(* Logix 5000 AddOnInstructionDefinition export SPEL_Above; software revision 30.01; part 6 of 9 *)

ADD_ON_INSTRUCTION SPEL_MotorGet   (* revision 1.2, vendor SEIKO EPSON CORP. *)
// Gets the state of the motor.
VAR_INPUT
   Start : BOOL; {required}
END_VAR
VAR_OUTPUT
   InCycle : BOOL; {access None, visible}
END_VAR
VAR_IN_OUT
   ExtInputs : AB:ETHERNET_MODULE_INT_128Bytes:I:0; {required}
   ExtOutputs : AB:ETHERNET_MODULE_INT_128Bytes:O:0; {required}
END_VAR
VAR_OUTPUT
   ErrCode1 : INT; {access None, visible}
   ErrCode2 : INT; {access None, visible}
   Status : INT; {visible}
   Done : BOOL; {access Read Only, visible}
   Error : BOOL; {visible}
END_VAR
VAR
   ExecMotor : SPEL_ExecCmd := (MaxTime := 3000); {access None}
   ExecTimeout : DINT; {access None}
END_VAR

ROUTINE Logic   (* ladder *)
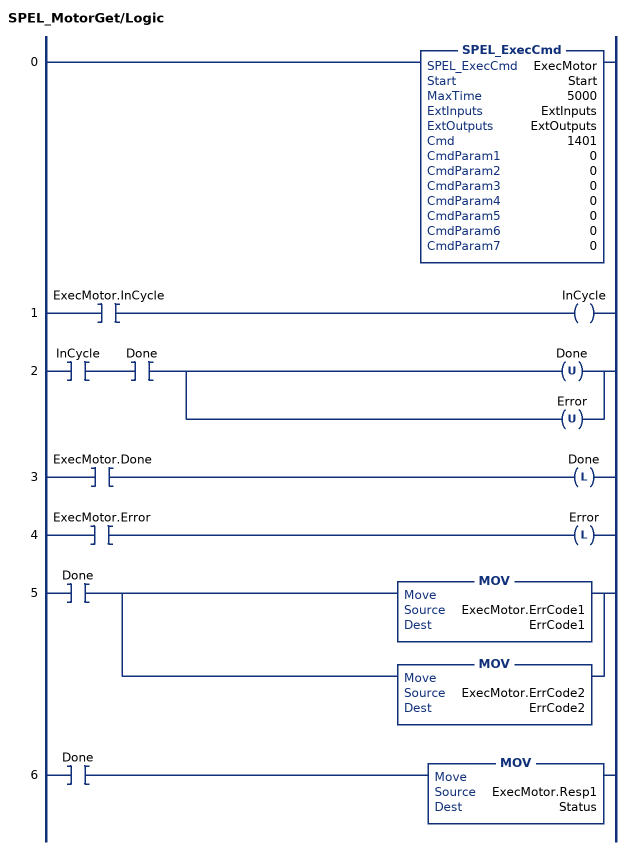
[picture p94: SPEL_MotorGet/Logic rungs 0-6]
   0: SPEL_ExecCmd(ExecMotor,Start,5000,ExtInputs,ExtOutputs,1401,0,0,0,0,0,0,0);
   1: XIC(ExecMotor.InCycle)OTE(InCycle);
   2: XIC(InCycle)XIC(Done)[OTU(Done) ,OTU(Error) ];
   3: XIC(ExecMotor.Done)OTL(Done);
   4: XIC(ExecMotor.Error)OTL(Error);
   5: XIC(Done)[MOV(ExecMotor.ErrCode1,ErrCode1) ,MOV(ExecMotor.ErrCode2,ErrCode2) ];
   6: XIC(Done)MOV(ExecMotor.Resp1,Status);
END_ROUTINE
END_ADD_ON_INSTRUCTION

ADD_ON_INSTRUCTION SPEL_MotorOff   (* revision 1.0, vendor SEIKO EPSON CORP. *)
// Turns robot motors off.
VAR_INPUT
   Start : BOOL; {access Read Only, required}
END_VAR
VAR_OUTPUT
   InCycle : BOOL; {access Read Only, visible}
   Done : BOOL; {access Read Only, visible}
   Error : BOOL; {access Read Only, visible}
END_VAR
VAR_IN_OUT
   ExtInputs : AB:ETHERNET_MODULE_INT_128Bytes:I:0; {required}
   ExtOutputs : AB:ETHERNET_MODULE_INT_128Bytes:O:0; {required}
END_VAR
VAR_OUTPUT
   ErrCode1 : INT; {access Read Only, visible}
   ErrCode2 : INT; {access Read Only, visible}
END_VAR
VAR
   ExecMotorOff : SPEL_ExecCmd := (MaxTime := 3000); {access None}
        .INCYCLE   // ExecInCycle
        .DONE   // ExecDone
        .ERROR   // ExecError
   OneShotStart : BOOL; {access None}
   StartCoil : BOOL; {access None}
   ExecTimeout : DINT; {access None}
END_VAR

ROUTINE Logic   (* ladder *)
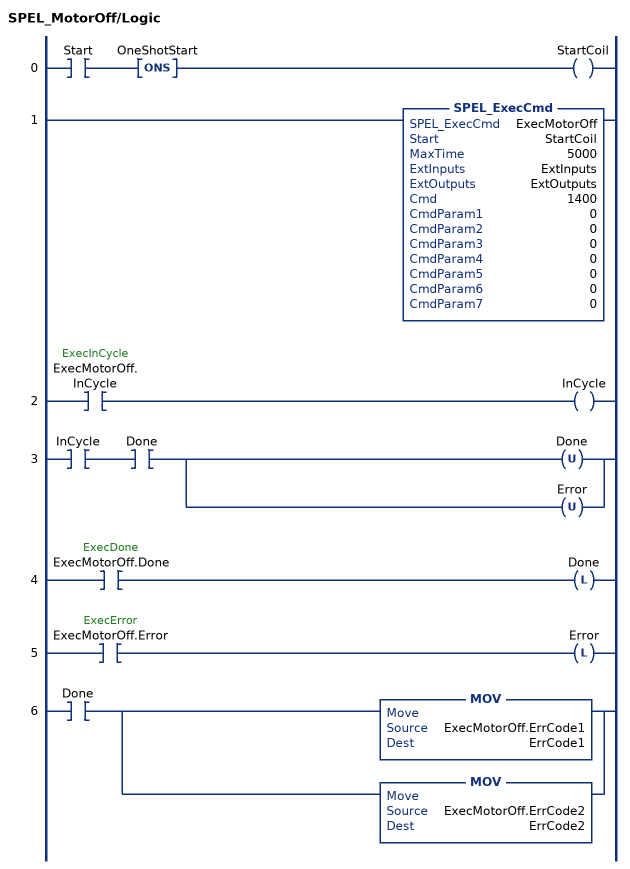
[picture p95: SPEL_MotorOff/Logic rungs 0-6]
   0: XIC(Start)ONS(OneShotStart)OTE(StartCoil);
   1: SPEL_ExecCmd(ExecMotorOff,StartCoil,5000,ExtInputs,ExtOutputs,1400,0,0,0,0,0,0,0);
   2: XIC(ExecMotorOff.InCycle)OTE(InCycle);
   3: XIC(InCycle)XIC(Done)[OTU(Done) ,OTU(Error) ];
   4: XIC(ExecMotorOff.Done)OTL(Done);
   5: XIC(ExecMotorOff.Error)OTL(Error);
   6: XIC(Done)[MOV(ExecMotorOff.ErrCode1,ErrCode1) ,MOV(ExecMotorOff.ErrCode2,ErrCode2) ];
END_ROUTINE
END_ADD_ON_INSTRUCTION

ADD_ON_INSTRUCTION SPEL_MotorOn   (* revision 1.0, vendor SEIKO EPSON CORP. *)
// Turns robot motors on.
VAR_INPUT
   Start : BOOL; {access Read Only, required}
END_VAR
VAR_OUTPUT
   InCycle : BOOL; {access Read Only, visible}
   Done : BOOL; {access Read Only, visible}
   Error : BOOL; {access Read Only, visible}
END_VAR
VAR_IN_OUT
   ExtInputs : AB:ETHERNET_MODULE_INT_128Bytes:I:0; {required}
   ExtOutputs : AB:ETHERNET_MODULE_INT_128Bytes:O:0; {required}
END_VAR
VAR_OUTPUT
   ErrCode1 : INT; {access Read Only, visible}
   ErrCode2 : INT; {access Read Only, visible}
END_VAR
VAR
   ExecMotorOn : SPEL_ExecCmd := (MaxTime := 3000); {access None}
        .INCYCLE   // ExecInCycle
        .DONE   // ExecDone
        .ERROR   // ExecError
   OneShotStart : BOOL; {access None}
   StartCoil : BOOL; {access None}
   ExecTimeout : DINT; {access None}
END_VAR

ROUTINE Logic   (* ladder *)
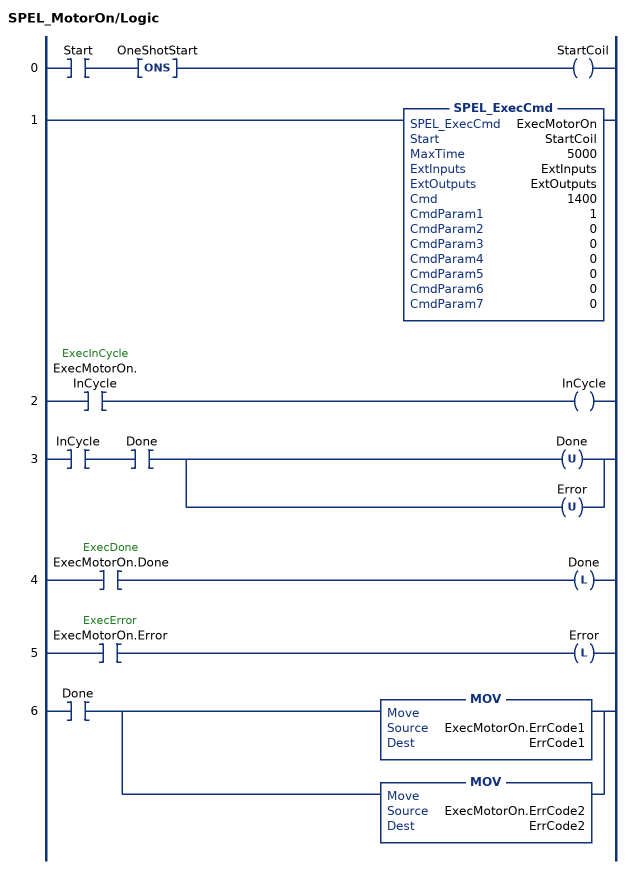
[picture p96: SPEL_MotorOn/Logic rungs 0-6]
   0: XIC(Start)ONS(OneShotStart)OTE(StartCoil);
   1: SPEL_ExecCmd(ExecMotorOn,StartCoil,5000,ExtInputs,ExtOutputs,1400,1,0,0,0,0,0,0);
   2: XIC(ExecMotorOn.InCycle)OTE(InCycle);
   3: XIC(InCycle)XIC(Done)[OTU(Done) ,OTU(Error) ];
   4: XIC(ExecMotorOn.Done)OTL(Done);
   5: XIC(ExecMotorOn.Error)OTL(Error);
   6: XIC(Done)[MOV(ExecMotorOn.ErrCode1,ErrCode1) ,MOV(ExecMotorOn.ErrCode2,ErrCode2) ];
END_ROUTINE
END_ADD_ON_INSTRUCTION

ADD_ON_INSTRUCTION SPEL_Move   (* revision 1.0, vendor SEIKO EPSON CORP. *)
// Moves the arm from the current position to the specified position in a linear interpolation motion.
VAR_OUTPUT
   InCycle : BOOL; {access Read Only, visible}
   Done : BOOL; {access Read Only, visible}
   Error : BOOL; {access Read Only, visible}
END_VAR
VAR_INPUT
   Start : BOOL; {required}
   MaxTime : DINT := 30000; {access None, visible}
   TargetType : INT; {access None, visible}
   Point : INT; {required}
   PalletNum : INT; {access None, visible}
   PalletPosOrCol : INT; {access None, visible}
   PalletRow : INT; {access None, visible}
END_VAR
VAR_IN_OUT
   ExtInputs : AB:ETHERNET_MODULE_INT_128Bytes:I:0; {required}
   ExtOutputs : AB:ETHERNET_MODULE_INT_128Bytes:O:0; {required}
END_VAR
VAR_OUTPUT
   ErrCode1 : INT; {access Read Only, visible}
   ErrCode2 : INT; {access Read Only, visible}
END_VAR
VAR
   ExecMove : SPEL_ExecCmd := (MaxTime := 3000); {access None}
   StartInit : BOOL; {access None}
   PointOrPalletNum : INT; {access None}
   MoveTargetType : DINT; {access None}
   OneShotStart : BOOL; {access None}
   ExecTimeout : DINT; {access None}
   OneShotCP : BOOL; {access None}
   LocalCP : DINT; {access None}
   CmdParam1 : DINT; {access None}
   TargetTypeError : BOOL; {access None}
   StartExec : BOOL; {access None}
   ExecuteCmd : BOOL; {access None}
   OneShotTargetType : BOOL; {access None}
END_VAR

ROUTINE Logic   (* ladder *)
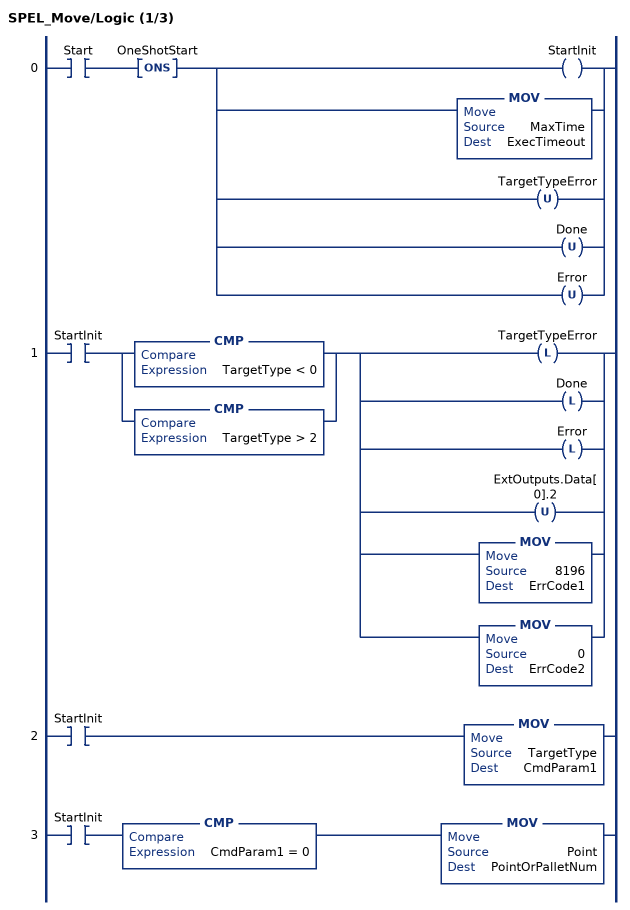
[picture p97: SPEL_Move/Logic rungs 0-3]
   0: XIC(Start)ONS(OneShotStart)[OTE(StartInit) ,MOV(MaxTime,ExecTimeout) ,OTU(TargetTypeError) ,OTU(Done) ,OTU(Error) ];
   1: XIC(StartInit)[CMP(TargetType < 0) ,CMP(TargetType > 2) ][OTL(TargetTypeError) ,OTL(Done) ,OTL(Error) ,OTU(ExtOutputs.Data[0].2) ,MOV(8196,ErrCode1) ,MOV(0,ErrCode2) ];
   2: XIC(StartInit)MOV(TargetType,CmdParam1);
   3: XIC(StartInit)CMP(CmdParam1 = 0)MOV(Point,PointOrPalletNum);
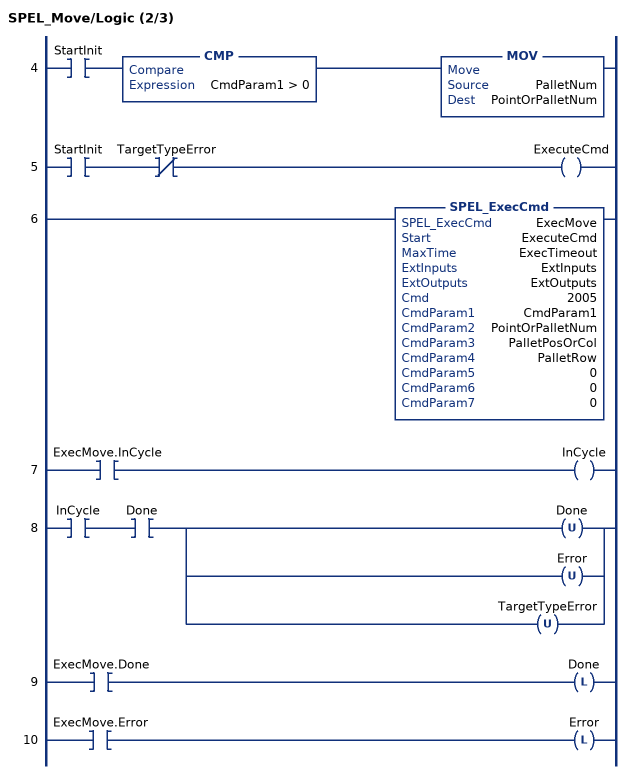
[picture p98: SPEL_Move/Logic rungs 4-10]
   4: XIC(StartInit)CMP(CmdParam1 > 0)MOV(PalletNum,PointOrPalletNum);
   5: XIC(StartInit)XIO(TargetTypeError)OTE(ExecuteCmd);
   6: SPEL_ExecCmd(ExecMove,ExecuteCmd,ExecTimeout,ExtInputs,ExtOutputs,2005,CmdParam1,PointOrPalletNum,PalletPosOrCol,PalletRow,0,0,0);
   7: XIC(ExecMove.InCycle)OTE(InCycle);
   8: XIC(InCycle)XIC(Done)[OTU(Done) ,OTU(Error) ,OTU(TargetTypeError) ];
   9: XIC(ExecMove.Done)OTL(Done);
   10: XIC(ExecMove.Error)OTL(Error);
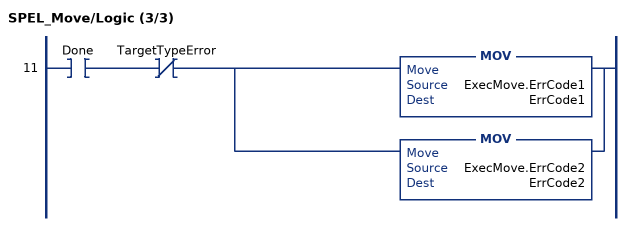
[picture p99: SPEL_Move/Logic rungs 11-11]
   11: XIC(Done)XIO(TargetTypeError)[MOV(ExecMove.ErrCode1,ErrCode1) ,MOV(ExecMove.ErrCode2,ErrCode2) ];
END_ROUTINE
END_ADD_ON_INSTRUCTION

ADD_ON_INSTRUCTION SPEL_NoFlip   (* revision 1.0, vendor SEIKO EPSON CORP. *)
// Sets the wrist orientation of the specified point to NOFLIP.
VAR_OUTPUT
   InCycle : BOOL; {access Read Only, visible}
   Done : BOOL; {access Read Only, visible}
   Error : BOOL; {access Read Only, visible}
END_VAR
VAR_INPUT
   Start : BOOL; {required}
   Point : INT; {required}
END_VAR
VAR_IN_OUT
   ExtInputs : AB:ETHERNET_MODULE_INT_128Bytes:I:0; {required}
   ExtOutputs : AB:ETHERNET_MODULE_INT_128Bytes:O:0; {required}
END_VAR
VAR_OUTPUT
   ErrCode1 : INT; {access Read Only, visible}
   ErrCode2 : INT; {access Read Only, visible}
END_VAR
VAR
   ExecNoFlip : SPEL_ExecCmd := (MaxTime := 3000); {access None}
   OneShotStart : BOOL; {access None}
   StartCoil : BOOL; {access None}
   ExecTimeout : DINT; {access None}
END_VAR

ROUTINE Logic   (* ladder *)
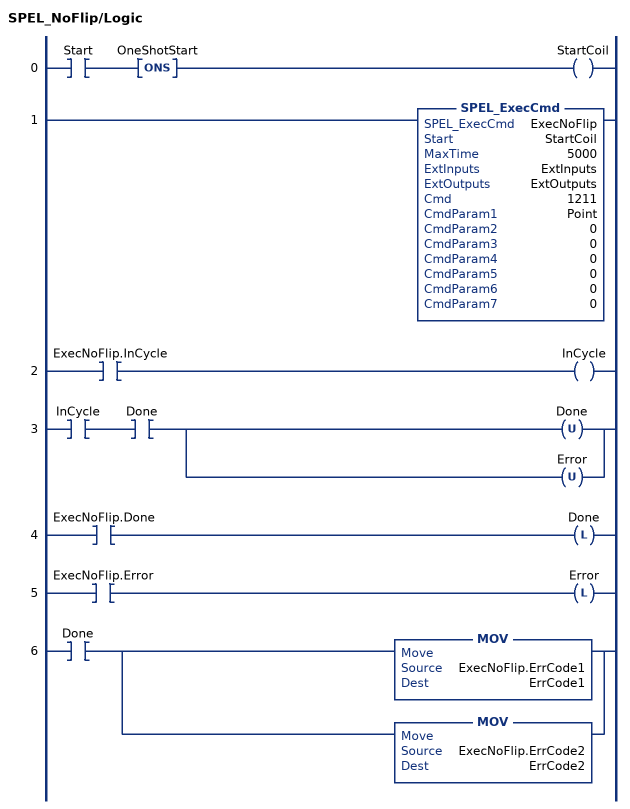
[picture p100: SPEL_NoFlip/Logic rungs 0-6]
   0: XIC(Start)ONS(OneShotStart)OTE(StartCoil);
   1: SPEL_ExecCmd(ExecNoFlip,StartCoil,5000,ExtInputs,ExtOutputs,1211,Point,0,0,0,0,0,0);
   2: XIC(ExecNoFlip.InCycle)OTE(InCycle);
   3: XIC(InCycle)XIC(Done)[OTU(Done) ,OTU(Error) ];
   4: XIC(ExecNoFlip.Done)OTL(Done);
   5: XIC(ExecNoFlip.Error)OTL(Error);
   6: XIC(Done)[MOV(ExecNoFlip.ErrCode1,ErrCode1) ,MOV(ExecNoFlip.ErrCode2,ErrCode2) ];
END_ROUTINE
END_ADD_ON_INSTRUCTION

ADD_ON_INSTRUCTION SPEL_Off   (* revision 1.0, vendor SEIKO EPSON CORP. *)
// Turns an output bit off.
VAR_OUTPUT
   InCycle : BOOL; {access Read Only, visible}
   Done : BOOL; {access Read Only, visible}
   Error : BOOL; {access Read Only, visible}
END_VAR
VAR_INPUT
   Start : BOOL; {access Read Only, required}
   Bit : INT; {required}
END_VAR
VAR_IN_OUT
   ExtInputs : AB:ETHERNET_MODULE_INT_128Bytes:I:0; {required}
   ExtOutputs : AB:ETHERNET_MODULE_INT_128Bytes:O:0; {required}
END_VAR
VAR_OUTPUT
   ErrCode1 : INT; {access Read Only, visible}
   ErrCode2 : INT; {access Read Only, visible}
END_VAR
VAR
   ExecOff : SPEL_ExecCmd := (MaxTime := 3000); {access None}
        .INCYCLE   // ExecInCycle
        .DONE   // ExecDone
        .ERROR   // ExecError
   OneShotStart : BOOL; {access None}
   StartCoil : BOOL; {access None}
   ExecTimeout : DINT; {access None}
END_VAR

ROUTINE Logic   (* ladder *)
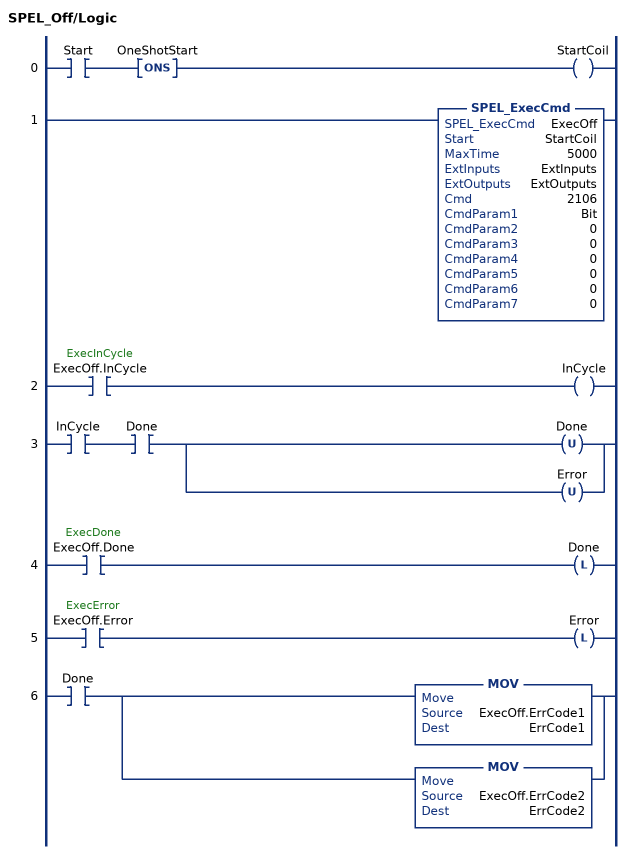
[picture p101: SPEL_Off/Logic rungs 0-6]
   0: XIC(Start)ONS(OneShotStart)OTE(StartCoil);
   1: SPEL_ExecCmd(ExecOff,StartCoil,5000,ExtInputs,ExtOutputs,2106,Bit,0,0,0,0,0,0);
   2: XIC(ExecOff.InCycle)OTE(InCycle);
   3: XIC(InCycle)XIC(Done)[OTU(Done) ,OTU(Error) ];
   4: XIC(ExecOff.Done)OTL(Done);
   5: XIC(ExecOff.Error)OTL(Error);
   6: XIC(Done)[MOV(ExecOff.ErrCode1,ErrCode1) ,MOV(ExecOff.ErrCode2,ErrCode2) ];
END_ROUTINE
END_ADD_ON_INSTRUCTION

ADD_ON_INSTRUCTION SPEL_On   (* revision 1.0, vendor SEIKO EPSON CORP. *)
// Turns an output bit on.
VAR_OUTPUT
   InCycle : BOOL; {access Read Only, visible}
   Done : BOOL; {access Read Only, visible}
   Error : BOOL; {access Read Only, visible}
END_VAR
VAR_INPUT
   Start : BOOL; {access Read Only, required}
   Bit : INT; {required}
END_VAR
VAR_IN_OUT
   ExtInputs : AB:ETHERNET_MODULE_INT_128Bytes:I:0; {required}
   ExtOutputs : AB:ETHERNET_MODULE_INT_128Bytes:O:0; {required}
END_VAR
VAR_OUTPUT
   ErrCode1 : INT; {access Read Only, visible}
   ErrCode2 : INT; {access Read Only, visible}
END_VAR
VAR
   ExecOn : SPEL_ExecCmd := (MaxTime := 3000); {access None}
        .INCYCLE   // ExecInCycle
        .DONE   // ExecDone
        .ERROR   // ExecError
   OneShotStart : BOOL; {access None}
   StartCoil : BOOL; {access None}
   ExecTimeout : DINT; {access None}
END_VAR

ROUTINE Logic   (* ladder *)
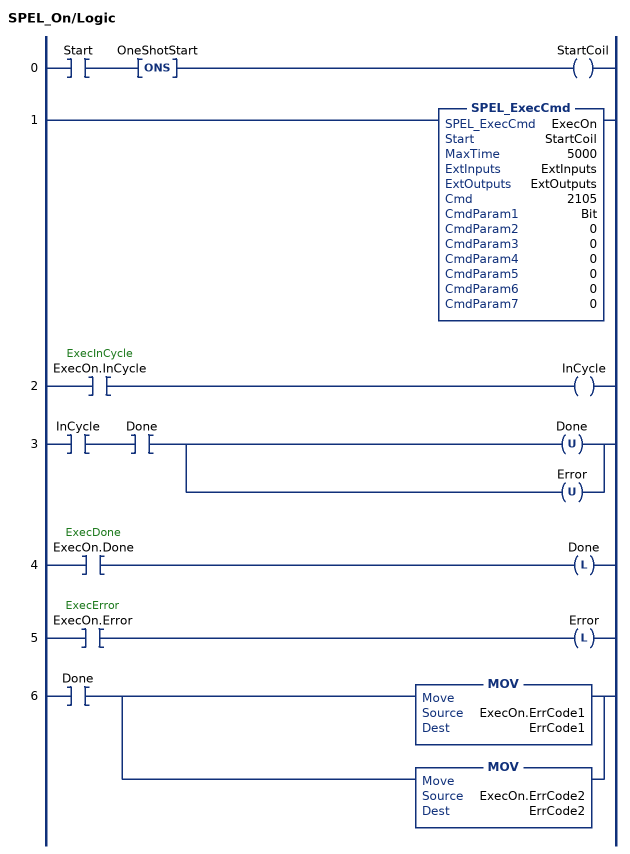
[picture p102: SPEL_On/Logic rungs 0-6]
   0: XIC(Start)ONS(OneShotStart)OTE(StartCoil);
   1: SPEL_ExecCmd(ExecOn,StartCoil,5000,ExtInputs,ExtOutputs,2105,Bit,0,0,0,0,0,0);
   2: XIC(ExecOn.InCycle)OTE(InCycle);
   3: XIC(InCycle)XIC(Done)[OTU(Done) ,OTU(Error) ];
   4: XIC(ExecOn.Done)OTL(Done);
   5: XIC(ExecOn.Error)OTL(Error);
   6: XIC(Done)[MOV(ExecOn.ErrCode1,ErrCode1) ,MOV(ExecOn.ErrCode2,ErrCode2) ];
END_ROUTINE
END_ADD_ON_INSTRUCTION

ADD_ON_INSTRUCTION SPEL_Oport   (* revision 1.2, vendor SEIKO EPSON CORP. *)
// Returns the state of the specified output bit.
VAR_INPUT
   Start : BOOL; {access None, required}
END_VAR
VAR_OUTPUT
   InCycle : BOOL; {access None, visible}
   Done : BOOL; {access Read Only, visible}
   Error : BOOL; {access None, visible}
END_VAR
VAR_INPUT
   BitNum : INT; {access None, required}
END_VAR
VAR_OUTPUT
   Status : INT; {access Read Only, visible}
END_VAR
VAR_IN_OUT
   ExtInputs : AB:ETHERNET_MODULE_INT_128Bytes:I:0; {required}
   ExtOutputs : AB:ETHERNET_MODULE_INT_128Bytes:O:0; {required}
END_VAR
VAR_OUTPUT
   ErrCode1 : INT; {access Read Only, visible}
   ErrCode2 : INT; {access Read Only, visible}
END_VAR
VAR
   ExecOport : SPEL_ExecCmd := (MaxTime := 3000); {access None}
END_VAR

ROUTINE Logic   (* ladder *)
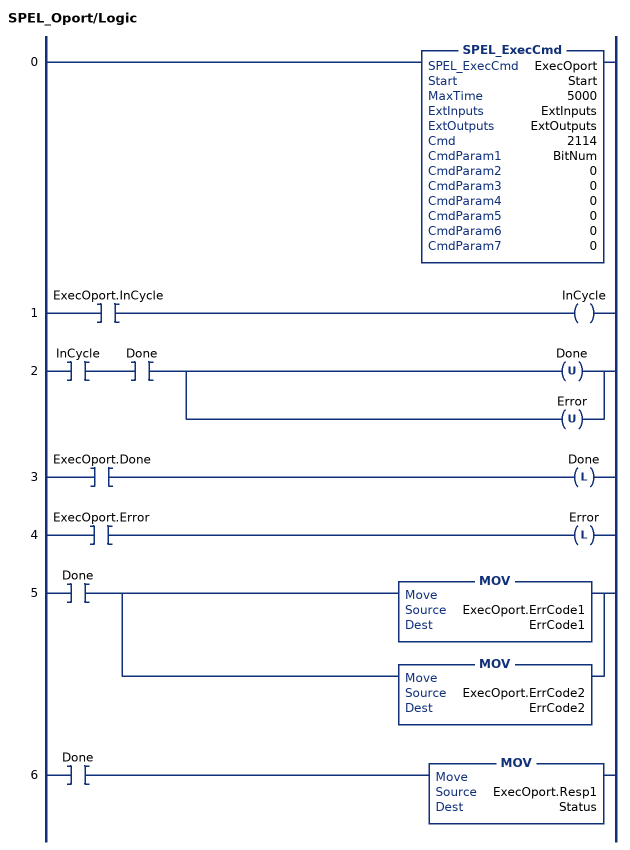
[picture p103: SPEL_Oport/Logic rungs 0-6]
   0: SPEL_ExecCmd(ExecOport,Start,5000,ExtInputs,ExtOutputs,2114,BitNum,0,0,0,0,0,0);
   1: XIC(ExecOport.InCycle)OTE(InCycle);
   2: XIC(InCycle)XIC(Done)[OTU(Done) ,OTU(Error) ];
   3: XIC(ExecOport.Done)OTL(Done);
   4: XIC(ExecOport.Error)OTL(Error);
   5: XIC(Done)[MOV(ExecOport.ErrCode1,ErrCode1) ,MOV(ExecOport.ErrCode2,ErrCode2) ];
   6: XIC(Done)MOV(ExecOport.Resp1,Status);
END_ROUTINE
END_ADD_ON_INSTRUCTION

ADD_ON_INSTRUCTION SPEL_Out   (* revision 1.0, vendor SEIKO EPSON CORP. *)
// Sets an output byte.
VAR_OUTPUT
   InCycle : BOOL; {access Read Only, visible}
   Done : BOOL; {access Read Only, visible}
   Error : BOOL; {access Read Only, visible}
END_VAR
VAR_INPUT
   Start : BOOL; {access Read Only, required}
   PortNum : INT; {required}
   OutData : INT; {required}
END_VAR
VAR_IN_OUT
   ExtInputs : AB:ETHERNET_MODULE_INT_128Bytes:I:0; {required}
   ExtOutputs : AB:ETHERNET_MODULE_INT_128Bytes:O:0; {required}
END_VAR
VAR_OUTPUT
   ErrCode1 : INT; {access Read Only, visible}
   ErrCode2 : INT; {access Read Only, visible}
END_VAR
VAR
   ExeOut : SPEL_ExecCmd := (MaxTime := 3000); {access None}
        .INCYCLE   // ExecInCycle
        .DONE   // ExecDone
        .ERROR   // ExecError
   OneShotStart : BOOL; {access None}
   StartCoil : BOOL; {access None}
   ExecTimeout : DINT; {access None}
END_VAR

ROUTINE Logic   (* ladder *)
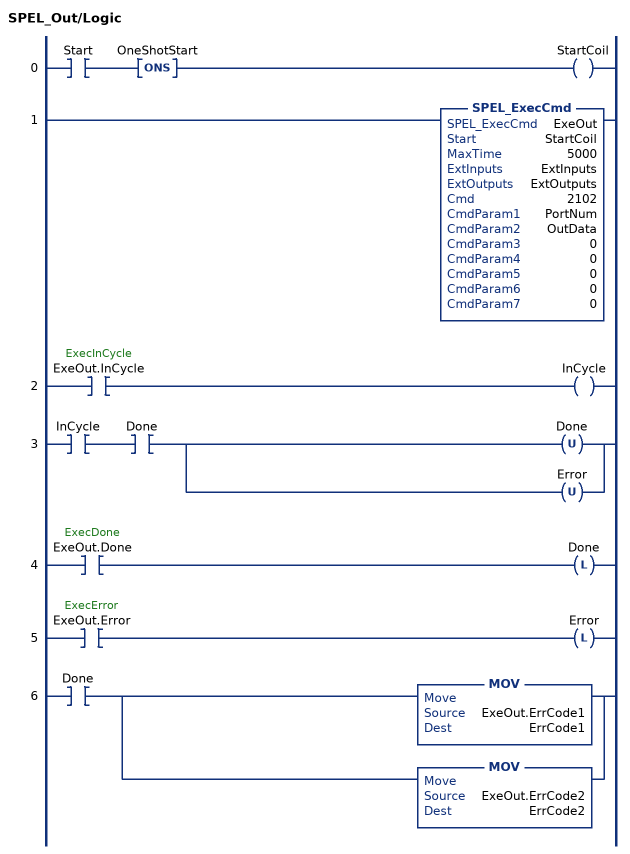
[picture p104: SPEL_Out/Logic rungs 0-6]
   0: XIC(Start)ONS(OneShotStart)OTE(StartCoil);
   1: SPEL_ExecCmd(ExeOut,StartCoil,5000,ExtInputs,ExtOutputs,2102,PortNum,OutData,0,0,0,0,0);
   2: XIC(ExeOut.InCycle)OTE(InCycle);
   3: XIC(InCycle)XIC(Done)[OTU(Done) ,OTU(Error) ];
   4: XIC(ExeOut.Done)OTL(Done);
   5: XIC(ExeOut.Error)OTL(Error);
   6: XIC(Done)[MOV(ExeOut.ErrCode1,ErrCode1) ,MOV(ExeOut.ErrCode2,ErrCode2) ];
END_ROUTINE
END_ADD_ON_INSTRUCTION

ADD_ON_INSTRUCTION SPEL_OutW   (* revision 1.0, vendor SEIKO EPSON CORP. *)
// Sets an output word.
VAR_OUTPUT
   InCycle : BOOL; {access Read Only, visible}
   Done : BOOL; {access Read Only, visible}
   Error : BOOL; {access Read Only, visible}
END_VAR
VAR_INPUT
   Start : BOOL; {access Read Only, required}
   PortNum : INT; {required}
   OutData : DINT; {required}
END_VAR
VAR_IN_OUT
   ExtInputs : AB:ETHERNET_MODULE_INT_128Bytes:I:0; {required}
   ExtOutputs : AB:ETHERNET_MODULE_INT_128Bytes:O:0; {required}
END_VAR
VAR_OUTPUT
   ErrCode1 : INT; {access Read Only, visible}
   ErrCode2 : INT; {access Read Only, visible}
END_VAR
VAR
   ExeOutW : SPEL_ExecCmd := (MaxTime := 3000); {access None}
        .INCYCLE   // ExecInCycle
        .DONE   // ExecDone
        .ERROR   // ExecError
   OneShotStart : BOOL; {access None}
   StartCoil : BOOL; {access None}
   ExecTimeout : DINT; {access None}
END_VAR

ROUTINE Logic   (* ladder *)
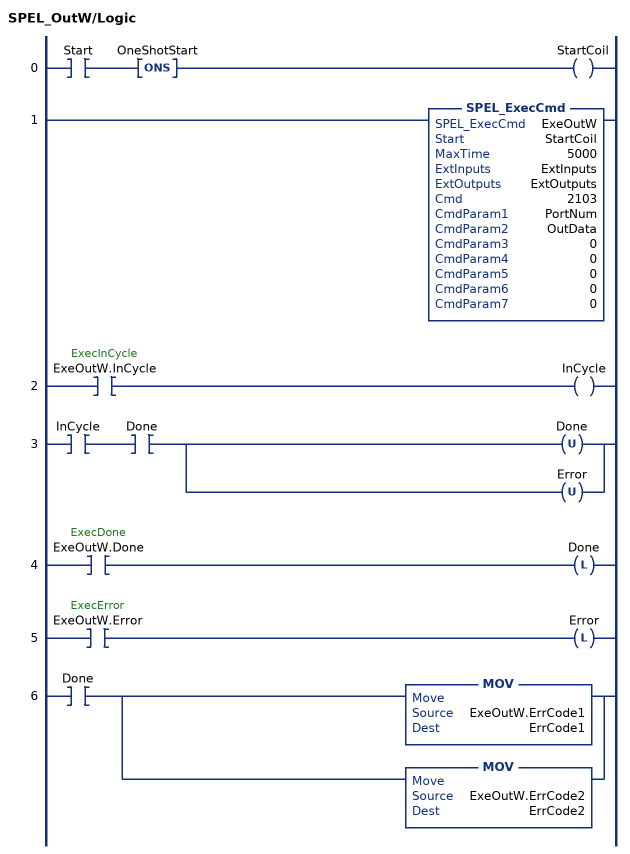
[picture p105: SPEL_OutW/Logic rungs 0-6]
   0: XIC(Start)ONS(OneShotStart)OTE(StartCoil);
   1: SPEL_ExecCmd(ExeOutW,StartCoil,5000,ExtInputs,ExtOutputs,2103,PortNum,OutData,0,0,0,0,0);
   2: XIC(ExeOutW.InCycle)OTE(InCycle);
   3: XIC(InCycle)XIC(Done)[OTU(Done) ,OTU(Error) ];
   4: XIC(ExeOutW.Done)OTL(Done);
   5: XIC(ExeOutW.Error)OTL(Error);
   6: XIC(Done)[MOV(ExeOutW.ErrCode1,ErrCode1) ,MOV(ExeOutW.ErrCode2,ErrCode2) ];
END_ROUTINE
END_ADD_ON_INSTRUCTION

ADD_ON_INSTRUCTION SPEL_Pallet3Get   (* revision 1.2, vendor SEIKO EPSON CORP. *)
// Acquires the details of 3-point definition of the specified pallet.
VAR_OUTPUT
   InCycle : BOOL; {access None, visible}
   Done : BOOL; {access None, visible}
   Error : BOOL; {access None, visible}
END_VAR
VAR_INPUT
   Start : BOOL; {access None, required}
   PalletNum : INT; {access None, required}
   Point1 : INT; {access Read Only, required}
   Point2 : INT; {access None, required}
   Point3 : INT; {access None, required}
END_VAR
VAR_OUTPUT
   Rows : INT; {access Read Only, visible}
   Columns : INT; {access Read Only, visible}
END_VAR
VAR_IN_OUT
   ExtInputs : AB:ETHERNET_MODULE_INT_128Bytes:I:0; {required}
   ExtOutputs : AB:ETHERNET_MODULE_INT_128Bytes:O:0; {required}
END_VAR
VAR_OUTPUT
   ErrCode1 : INT; {access None, visible}
   ErrCode2 : INT; {access None, visible}
END_VAR
VAR
   ExecGetPallet : SPEL_ExecCmd := (MaxTime := 3000); {access None}
   ExecTimeout : DINT; {access None}
END_VAR

ROUTINE Logic   (* ladder *)
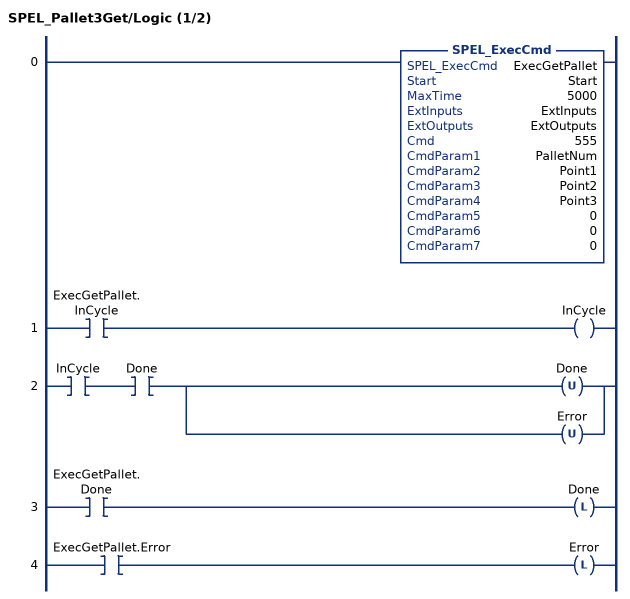
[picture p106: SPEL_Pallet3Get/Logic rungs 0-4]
   0: SPEL_ExecCmd(ExecGetPallet,Start,5000,ExtInputs,ExtOutputs,555,PalletNum,Point1,Point2,Point3,0,0,0);
   1: XIC(ExecGetPallet.InCycle)OTE(InCycle);
   2: XIC(InCycle)XIC(Done)[OTU(Done) ,OTU(Error) ];
   3: XIC(ExecGetPallet.Done)OTL(Done);
   4: XIC(ExecGetPallet.Error)OTL(Error);
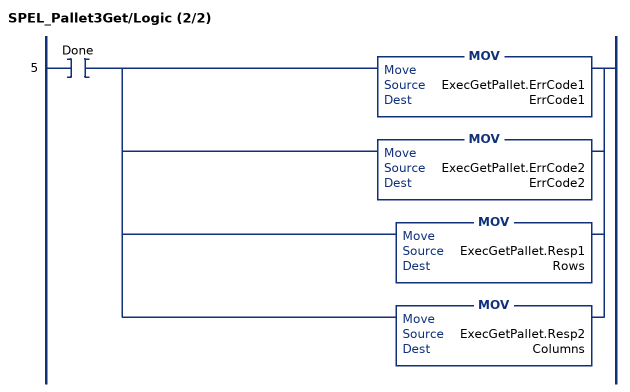
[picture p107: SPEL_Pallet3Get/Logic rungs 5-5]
   5: XIC(Done)[MOV(ExecGetPallet.ErrCode1,ErrCode1) ,MOV(ExecGetPallet.ErrCode2,ErrCode2) ,MOV(ExecGetPallet.Resp1,Rows) ,MOV(ExecGetPallet.Resp2,Columns) ];
END_ROUTINE
END_ADD_ON_INSTRUCTION

ADD_ON_INSTRUCTION SPEL_Pallet3Set   (* revision 1.0, vendor SEIKO EPSON CORP. *)
// Defines a pallet by specifying 3 points.
VAR_OUTPUT
   InCycle : BOOL; {access Read Only, visible}
   Done : BOOL; {access Read Only, visible}
   Error : BOOL; {access Read Only, visible}
END_VAR
VAR_INPUT
   Start : BOOL; {required}
   PalletNum : INT; {access None, required}
   Point1 : INT; {required}
   Point2 : INT; {required}
   Point3 : INT; {required}
   Columns : INT; {access None, required}
   Rows : INT; {access None, required}
END_VAR
VAR_IN_OUT
   ExtInputs : AB:ETHERNET_MODULE_INT_128Bytes:I:0; {required}
   ExtOutputs : AB:ETHERNET_MODULE_INT_128Bytes:O:0; {required}
END_VAR
VAR_OUTPUT
   ErrCode1 : INT; {access Read Only, visible}
   ErrCode2 : INT; {access Read Only, visible}
END_VAR
VAR
   ExecSetPallet : SPEL_ExecCmd := (MaxTime := 3000); {access None}
   StartInit : BOOL; {access None}
   OneShotStart : BOOL; {access None}
   ExecTimeout : DINT; {access None}
END_VAR

ROUTINE Logic   (* ladder *)
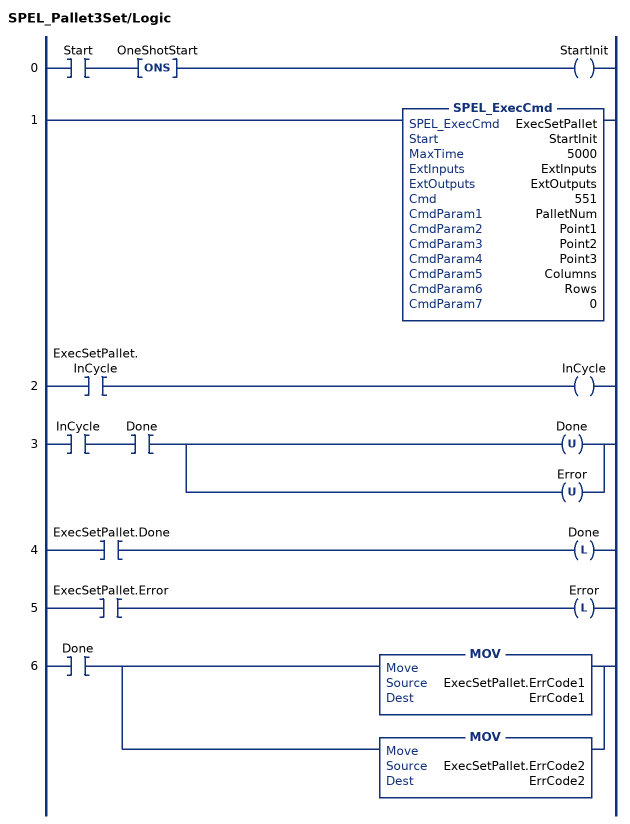
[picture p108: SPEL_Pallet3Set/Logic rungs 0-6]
   0: XIC(Start)ONS(OneShotStart)OTE(StartInit);
   1: SPEL_ExecCmd(ExecSetPallet,StartInit,5000,ExtInputs,ExtOutputs,551,PalletNum,Point1,Point2,Point3,Columns,Rows,0);
   2: XIC(ExecSetPallet.InCycle)OTE(InCycle);
   3: XIC(InCycle)XIC(Done)[OTU(Done) ,OTU(Error) ];
   4: XIC(ExecSetPallet.Done)OTL(Done);
   5: XIC(ExecSetPallet.Error)OTL(Error);
   6: XIC(Done)[MOV(ExecSetPallet.ErrCode1,ErrCode1) ,MOV(ExecSetPallet.ErrCode2,ErrCode2) ];
END_ROUTINE
END_ADD_ON_INSTRUCTION

ADD_ON_INSTRUCTION SPEL_Pallet4Get   (* revision 1.2, vendor SEIKO EPSON CORP. *)
// Acquires the details of 4-point definition of the specified pallet.
VAR_OUTPUT
   InCycle : BOOL; {access None, visible}
   Done : BOOL; {access None, visible}
   Error : BOOL; {access None, visible}
END_VAR
VAR_INPUT
   Start : BOOL; {access None, required}
   PalletNum : INT; {access None, required}
   Point1 : INT; {access Read Only, required}
   Point2 : INT; {access None, required}
   Point3 : INT; {access None, required}
   Point4 : INT; {access Read Only, required}
END_VAR
VAR_OUTPUT
   Rows : INT; {access Read Only, visible}
   Columns : INT; {access Read Only, visible}
END_VAR
VAR_IN_OUT
   ExtInputs : AB:ETHERNET_MODULE_INT_128Bytes:I:0; {required}
   ExtOutputs : AB:ETHERNET_MODULE_INT_128Bytes:O:0; {required}
END_VAR
VAR_OUTPUT
   ErrCode1 : INT; {access None, visible}
   ErrCode2 : INT; {access None, visible}
END_VAR
VAR
   ExecGetPallet : SPEL_ExecCmd := (MaxTime := 3000); {access None}
   ExecTimeout : DINT; {access None}
   CmdParam2 : INT; {access None}
   CmdParam3 : INT; {access None}
   CmdParam4 : INT; {access None}
   CmdParam5 : INT; {access None}
   CmdParam6 : INT; {access None}
   CmdParam7 : INT; {access None}
END_VAR

ROUTINE Logic   (* ladder *)
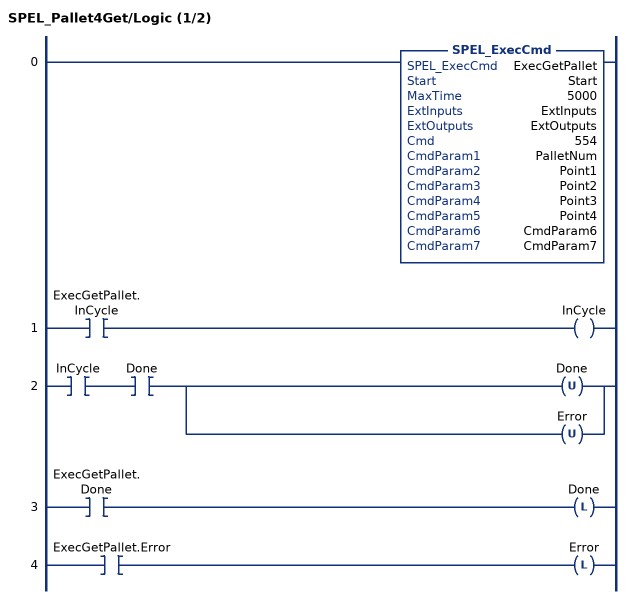
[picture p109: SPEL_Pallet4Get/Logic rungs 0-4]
   0: SPEL_ExecCmd(ExecGetPallet,Start,5000,ExtInputs,ExtOutputs,554,PalletNum,Point1,Point2,Point3,Point4,CmdParam6,CmdParam7);
   1: XIC(ExecGetPallet.InCycle)OTE(InCycle);
   2: XIC(InCycle)XIC(Done)[OTU(Done) ,OTU(Error) ];
   3: XIC(ExecGetPallet.Done)OTL(Done);
   4: XIC(ExecGetPallet.Error)OTL(Error);
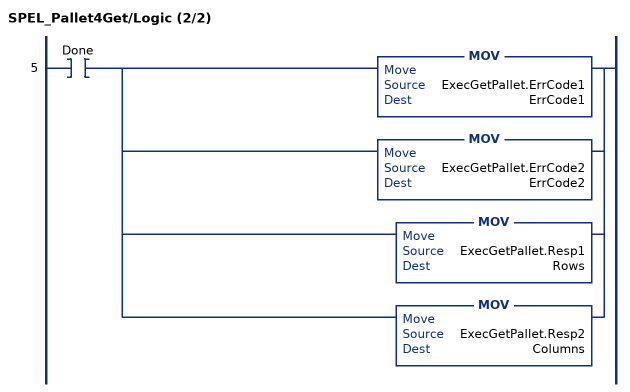
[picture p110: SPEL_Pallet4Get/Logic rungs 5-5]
   5: XIC(Done)[MOV(ExecGetPallet.ErrCode1,ErrCode1) ,MOV(ExecGetPallet.ErrCode2,ErrCode2) ,MOV(ExecGetPallet.Resp1,Rows) ,MOV(ExecGetPallet.Resp2,Columns) ];
END_ROUTINE
END_ADD_ON_INSTRUCTION

ADD_ON_INSTRUCTION SPEL_Pallet4Set   (* revision 1.0, vendor SEIKO EPSON CORP. *)
// Defines a pallet by specifying 4 points.
VAR_OUTPUT
   InCycle : BOOL; {access Read Only, visible}
   Done : BOOL; {access Read Only, visible}
   Error : BOOL; {access Read Only, visible}
END_VAR
VAR_INPUT
   Start : BOOL; {required}
   PalletNum : INT; {access None, required}
   Point1 : DINT; {required}
   Point2 : DINT; {required}
   Point3 : DINT; {required}
   Point4 : INT; {access None, required}
   Columns : INT; {access None, required}
   Rows : INT; {access None, required}
END_VAR
VAR_IN_OUT
   ExtInputs : AB:ETHERNET_MODULE_INT_128Bytes:I:0; {required}
   ExtOutputs : AB:ETHERNET_MODULE_INT_128Bytes:O:0; {required}
END_VAR
VAR_OUTPUT
   ErrCode1 : INT; {access Read Only, visible}
   ErrCode2 : INT; {access Read Only, visible}
END_VAR
VAR
   ExecSetPallet : SPEL_ExecCmd := (MaxTime := 3000); {access None}
   StartInit : BOOL; {access None}
   OneShotStart : BOOL; {access None}
   ExecTimeout : DINT; {access None}
END_VAR

ROUTINE Logic   (* ladder *)
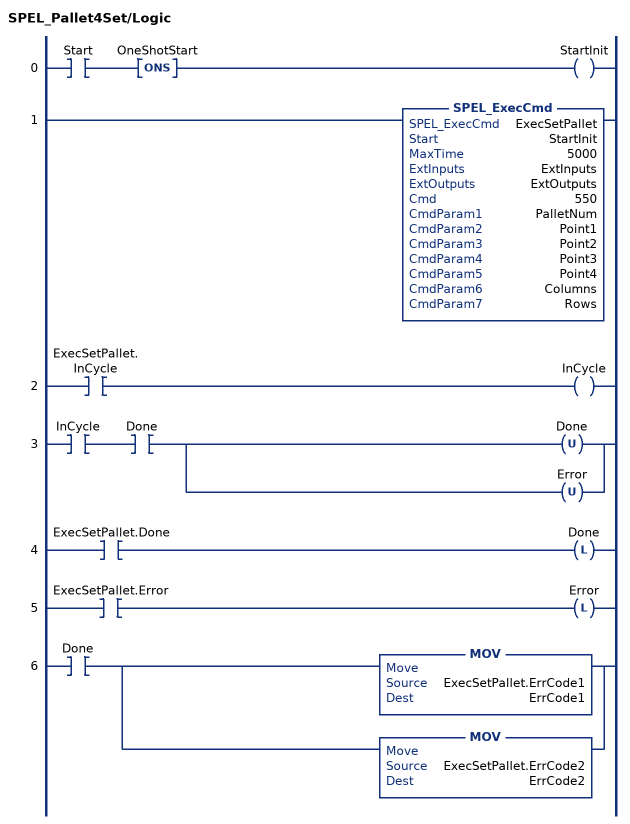
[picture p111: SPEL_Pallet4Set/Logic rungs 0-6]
   0: XIC(Start)ONS(OneShotStart)OTE(StartInit);
   1: SPEL_ExecCmd(ExecSetPallet,StartInit,5000,ExtInputs,ExtOutputs,550,PalletNum,Point1,Point2,Point3,Point4,Columns,Rows);
   2: XIC(ExecSetPallet.InCycle)OTE(InCycle);
   3: XIC(InCycle)XIC(Done)[OTU(Done) ,OTU(Error) ];
   4: XIC(ExecSetPallet.Done)OTL(Done);
   5: XIC(ExecSetPallet.Error)OTL(Error);
   6: XIC(Done)[MOV(ExecSetPallet.ErrCode1,ErrCode1) ,MOV(ExecSetPallet.ErrCode2,ErrCode2) ];
END_ROUTINE
END_ADD_ON_INSTRUCTION
